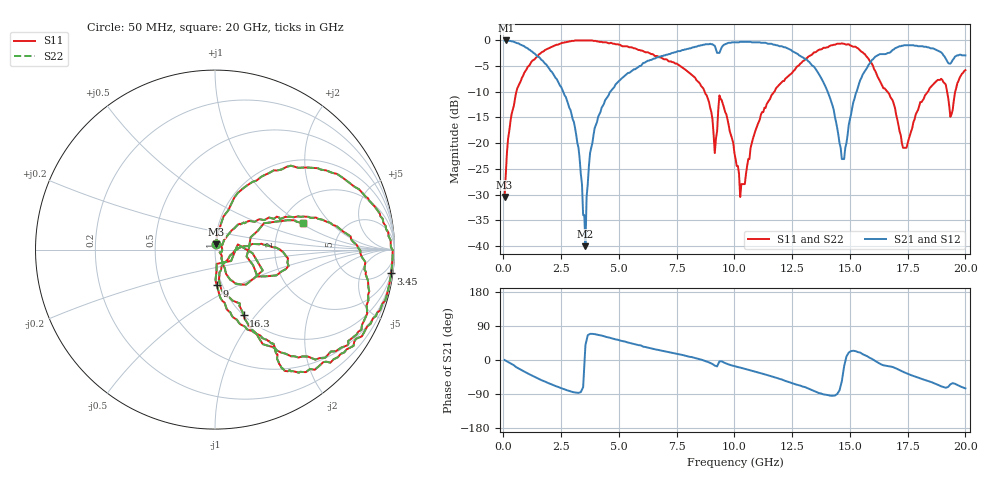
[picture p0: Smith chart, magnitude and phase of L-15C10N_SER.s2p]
# MHZ S MA R 50
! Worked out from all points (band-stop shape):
!   400 points, 50 MHz to 20 GHz, reference 50 ohm
!   highest |S21| = -0.09 dB at 100 MHz (marker M1); lowest = -40.0 dB at 3.55 GHz (marker M2)
!   |S21| within 3 dB of the highest: 6.904 GHz to 12.85 GHz (5.941 GHz wide, 60.2 % of centre); 16.15 GHz to 19.07 GHz (2.918 GHz wide, 16.6 % of centre)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
!   lowest |S11| = -30.5 dB at 50 MHz (marker M3), VSWR 1.06, Z = 50.6 + j2.96 ohm
!   |S11| at or under -10 dB: start of sweep to 560.8 MHz; 8.709 GHz to 11.73 GHz (3.022 GHz wide, 29.6 % of centre); 16.62 GHz to 18.38 GHz (1.763 GHz wide, 10.1 % of centre)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
!   |S22| runs from -30.5 to -0.1 dB; largest |S21 - S12| = 0
!   S11 on the Smith chart (normalised r, x): 50 MHz: 1.01, +0.06; 3.45 GHz: 1, -15; 9 GHz: 0.94, -0.39; 16.3 GHz: 1.00, -0.87; 20 GHz: 2.60, +1.05
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50  0.03 77.4  0.99 -0.1  0.99 -0.1  0.03 77.4
100  0.05 79.4  0.99 -1.9  0.99 -1.9  0.05 79.4
1050  0.55 53.4  0.83 -35.5  0.83 -35.5  0.55 53.4
2700  0.95 9.1  0.28 -78.7  0.28 -78.7  0.95 9.1
3400  0.99 -6.5  0.04 -78.1  0.04 -78.1  0.99 -6.5
3450  0.99 -7.7  0.02 -71.6  0.02 -71.6  0.99 -7.7
3550  0.99 -10.0  0.01 39.6  0.01 39.6  0.99 -10.0
3750  0.99 -14.5  0.08 69.0  0.08 69.0  0.99 -14.5
4100  0.97 -22.4  0.18 66.3  0.18 66.3  0.97 -22.4
6700  0.69 -59.8  0.68 26.6  0.68 26.6  0.69 -59.8
9000  0.2 -87.3  0.91 -9.2  0.91 -9.2  0.2 -87.3
9150  0.08 -83.3  0.88 -14.8  0.88 -14.8  0.08 -83.3
9350  0.29 -23.6  0.75 -3.6  0.75 -3.6  0.29 -23.6
10050  0.07 -56.4  0.95 -16.9  0.95 -16.9  0.07 -56.4
10250  0.03 -29.9  0.96 -20.0  0.96 -20.0  0.03 -29.9
11200  0.2 46.1  0.94 -35.9  0.94 -35.9  0.2 46.1
13350  0.72 8.1  0.57 -79.3  0.57 -79.3  0.72 8.1
14750  0.92 -30.9  0.07 -16.4  0.07 -16.4  0.92 -30.9
16300  0.4 -66.5  0.73 -9.8  0.73 -9.8  0.4 -66.5
16700  0.3 -71.0  0.75 -16.7  0.75 -16.7  0.3 -71.0
17450  0.09 -21.2  0.89 -35.1  0.89 -35.1  0.09 -21.2
20000  0.51 17.0  0.71 -74.9  0.71 -74.9  0.51 17.0
